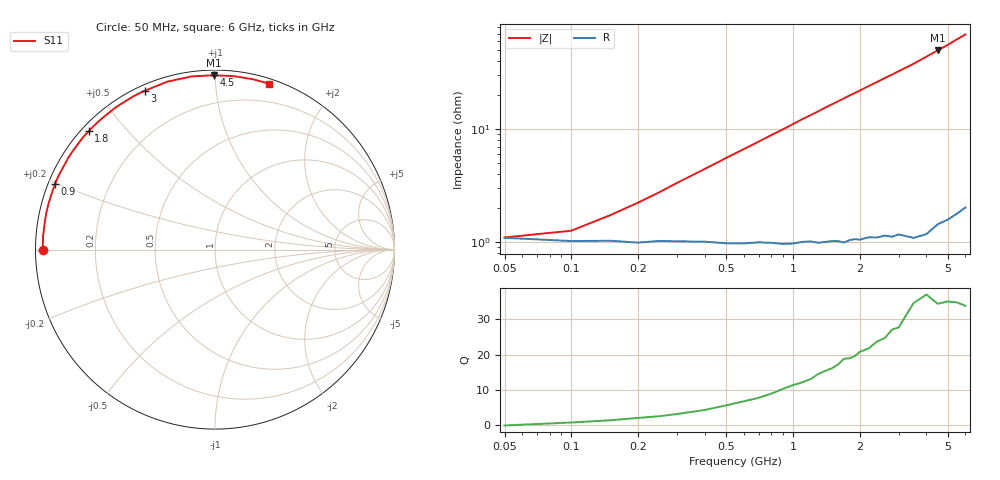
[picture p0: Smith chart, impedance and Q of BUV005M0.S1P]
! Infineon Technologies  Discrete & RF Semiconductors
! BB 833
! Si Tuning Diode in SOD323
! VR =
! S-Parameters:  June  1999
# GHz  S  MA  R  50
!  f  S11
! GHz  MAG  ANG
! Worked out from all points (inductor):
!   34 points, 50 MHz to 6 GHz, reference 50 ohm
!   read as one part to ground: L = 1.72 nH near 300 MHz
!   highest Q = 35.1 at 4.5 GHz (marker M1), where L = 1.76 nH
!   S11 on the Smith chart (normalised r, x): 50 MHz: 0.02, -0.00; 900 MHz: 0.02, +0.20; 1.8 GHz: 0.02, +0.40; 3 GHz: 0.02, +0.65; 4.5 GHz: 0.03, +0.99; 6 GHz: 0.04, +1.37
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0.05  0.9572 -179.7
0.1  0.9598 178.3
0.2  0.9611 175.4
0.25  0.9598 174.1
0.3  0.9602 172.7
0.5  0.962 167.5
0.6  0.9624 165.0
0.8  0.9624 160.0
0.9  0.9635 157.6
1  0.9635 155.1
1.1  0.9627 152.6
1.3  0.9641 148.0
1.4  0.9639 145.6
1.6  0.9643 141.2
1.7  0.9657 139.0
1.8  0.9645 136.8
2  0.9652 132.7
2.2  0.9648 128.6
2.4  0.966 124.8
2.6  0.9659 121.0
2.8  0.9678 117.5
3  0.9676 113.9
3.5  0.9726 105.8
4  0.9736 97.7
4.5  0.9714 90.4
5  0.972 83.9
5.5  0.9723 77.5
6  0.9723 72.1
